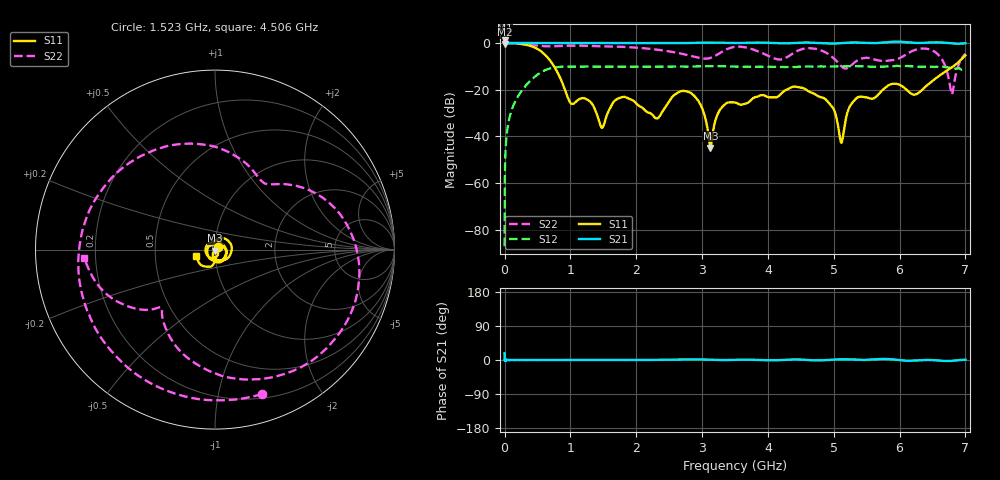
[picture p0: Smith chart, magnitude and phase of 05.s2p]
!Keysight Technologies,N5232A,MY52221221,A.10.65.11
!Date: Wednesday, October 16, 2024 11:53:23
!Correction: S11(Full 2 Port(1,4))
!S41(Full 2 Port(1,4))
!S14(Full 2 Port(1,4))
!S44(Full 2 Port(1,4))
!S2P File: Measurements: S11, S41, S14, S44:
# Hz S  RI  R 50
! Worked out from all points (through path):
!   4001 points, 300 kHz to 7 GHz, reference 50 ohm
!   highest |S21| = 1.09 dB at 300 kHz (marker M1); lowest = -0.6 dB at 2.05 MHz (marker M2)
!   lowest |S11| = -44.9 dB at 3.127 GHz (marker M3), VSWR 1.01, Z = 50.1 - j0.561 ohm
!   |S11| at or under -10 dB: 750.9 MHz to 6.816 GHz (6.066 GHz wide, 160 % of centre)
!   |S22| runs from -22.1 to 0.0 dB; largest |S21 - S12| = 1.4
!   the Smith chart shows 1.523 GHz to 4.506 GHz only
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300000  -0.9926 -0.0146  1.08 0.345  -3.13e-07 4.42e-05  -0.9897 -0.0227
2049925  -0.9693 0.1503  0.9303 -0.0295  0.000139 0.000634  -0.9776 0.0976
7.204692e7  -0.8181 0.5692  0.9943 -0.00134  0.0118 0.0215  -0.9676 0.2344
2.015414e8  0.1377 0.9619  1.001 -0.000256  0.0701 0.0121  -0.7703 0.5938
3.415354e8  0.8923 0.1664  0.9998 -9.71e-05  0.0873 -0.0978  -0.4304 0.8299
4.867792e8  0.2819 -0.7087  1 -0.000561  -0.0803 -0.1877  -0.0497 0.8795
6.320229e8  -0.4584 -0.2606  0.998 0.00118  -0.2681 0.00988  0.2712 0.8052
1.1675e9  0.0301 0.0582  0.9984 0.0033  0.1665 -0.264  0.8457 -0.218
1.478987e9  0.0152 0.00132  0.9987 0.00223  -0.3117 0.0119  0.3575 -0.7704
1.687228e9  0.0603 -0.00204  0.9978 0.00223  -0.0325 0.3094  -0.1263 -0.8271
2.3347e9  -0.0013 0.0249  0.9907 0.0066  -0.2828 -0.1297  -0.641 0.3181
2.81068e9  0.0775 -0.0407  1 0.0233  0.2921 0.115  0.1065 0.5268
3.127416e9  0.000834 -0.0056  1.02 0.0128  -0.0601 -0.3126  0.3113 0.3636
3.50015e9  -0.0527 0.00608  0.9985 0.00635  -0.1285 0.2846  0.7934 -0.2388
3.792387e9  0.0654 -0.0185  1.018 0.00881  0.312 0.0134  0.0652 -0.7107
4.264867e9  -0.0231 -0.0942  0.9863 0.00678  -0.3037 -0.00876  -0.3414 -0.3311
4.66735e9  -0.0842 0.0163  1.016 -0.0117  0.2781 0.1426  -0.6132 0.4625
5.115331e9  0.00678 -0.00266  0.9922 0.0339  -0.2605 -0.178  0.1759 0.2633
5.83455e9  -0.0867 0.0893  1.044 0.0456  0.1329 -0.2865  0.3918 -0.1538
6.496022e9  0.00626 0.152  1.028 -0.00674  0.2726 0.1475  -0.6358 -0.2784
6.793509e9  0.288 -0.0827  0.9766 -0.0379  -0.0336 -0.2986  -0.0788 -0.000737
7e9  -0.4433 -0.3186  0.9897 0.0155  -0.2488 0.0498  -0.5884 -0.0416
